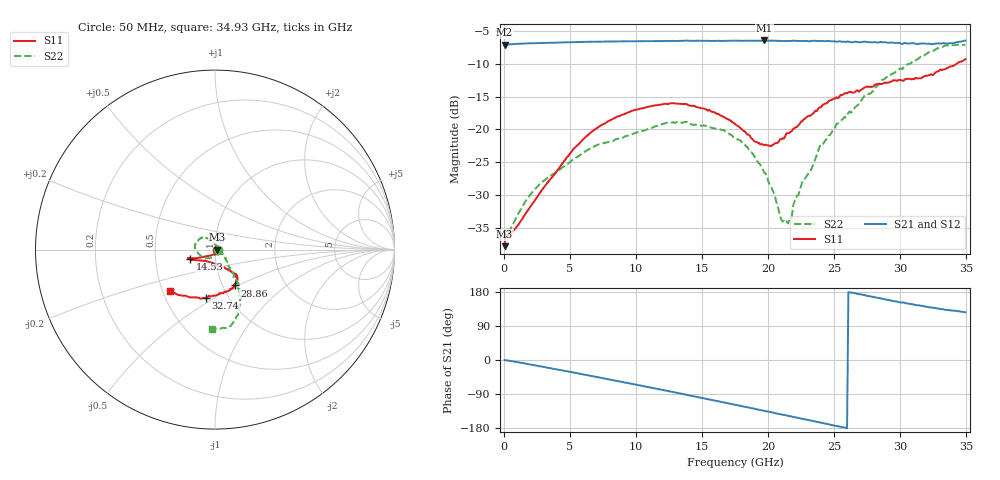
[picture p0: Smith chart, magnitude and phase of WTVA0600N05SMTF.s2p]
! 50 ohm 2-Port S-parameters measured by Modelithics Inc support@modelithics.com  Tampa, FL USA 813-866-6335 (February 2024)
! Smiths Interconnect,  6dB P/N: WTVA0600N05SMTF, Temperature: 0 C
! Board: 10 mil Rogers 4350B, Mounting Pad Dimensions: Length: 15 mils, Width: 25 mils, Gap: 40 mils.
# Hz S RI R 50
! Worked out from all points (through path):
!   352 points, 50 MHz to 34.93 GHz, reference 50 ohm
!   highest |S21| = -6.46 dB at 19.7 GHz (marker M1); lowest = -7.1 dB at 50 MHz (marker M2)
!   group delay of S21, straight-line fit = 19.4 ps
!   lowest |S11| = -37.8 dB at 50 MHz (marker M3), VSWR 1.03, Z = 51.3 - j0.0784 ohm
!   |S11| at or under -10 dB: start of sweep to 34.27 GHz
!   |S22| runs from -36.4 to -7.1 dB; largest |S21 - S12| = 0.003
!   S11 on the Smith chart (normalised r, x): 50 MHz: 1.03, -0.00; 14.53 GHz: 0.75, -0.08; 28.86 GHz: 1.14, -0.48; 32.74 GHz: 0.78, -0.46; 34.93 GHz: 0.54, -0.28
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5e7  0.0129 -0.000764  0.4412 -0.00136  0.4411 -0.00168  0.0164 -0.000587
1e8  0.0154 -0.00255  0.4415 -0.00319  0.4413 -0.0032  0.0147 -0.00359
8.965e8  0.0069 -0.0164  0.4457 -0.0376  0.4455 -0.0377  0.00773 -0.0196
2.6875e9  -0.0135 -0.0296  0.4361 -0.1264  0.4358 -0.1264  -0.00533 -0.0379
5.8715e9  -0.0702 -0.0417  0.3694 -0.2793  0.3692 -0.2793  -0.043 -0.0488
8.558e9  -0.1156 -0.048  0.2667 -0.3839  0.2662 -0.3839  -0.0761 -0.0378
1.1742e10  -0.1471 -0.0466  0.104 -0.4584  0.1033 -0.4583  -0.108 0.00144
1.4528e10  -0.1384 -0.0537  -0.0566 -0.4695  -0.057 -0.4692  -0.0983 0.0467
1.7513e10  -0.092 -0.0593  -0.2248 -0.4175  -0.2251 -0.4172  -0.0558 0.067
1.88065e10  -0.0559 -0.0633  -0.2897 -0.3752  -0.2896 -0.375  -0.0344 0.0563
1.9702e10  -0.0299 -0.0699  -0.3311 -0.341  -0.3307 -0.341  -0.0159 0.0441
2.0498e10  -0.00589 -0.078  -0.3632 -0.3038  -0.3634 -0.3032  -0.000812 0.0317
2.09955e10  0.00958 -0.0835  -0.38 -0.2789  -0.38 -0.2785  0.00875 0.0187
2.1493e10  0.0229 -0.0906  -0.3943 -0.2563  -0.3943 -0.2559  0.0161 0.0107
2.25875e10  0.0549 -0.1017  -0.4275 -0.1976  -0.4274 -0.1972  0.0373 -0.0152
2.33835e10  0.072 -0.11  -0.4455 -0.1564  -0.4453 -0.1561  0.047 -0.0253
2.3881e10  0.0862 -0.1193  -0.4551 -0.1237  -0.4549 -0.1236  0.0583 -0.0453
2.51745e10  0.1088 -0.1381  -0.4631 -0.0483  -0.4629 -0.0481  0.0759 -0.0801
2.8856e10  0.1093 -0.1997  -0.4327 0.1574  -0.4323 0.1581  0.1319 -0.2062
2.91545e10  0.1045 -0.2026  -0.4231 0.1713  -0.4226 0.1718  0.13 -0.2178
3.27365e10  -0.0517 -0.2695  -0.3267 0.3105  -0.327 0.3099  0.1138 -0.3946
3.49255e10  -0.2521 -0.2308  -0.2776 0.384  -0.2758 0.385  -0.0183 -0.4424
